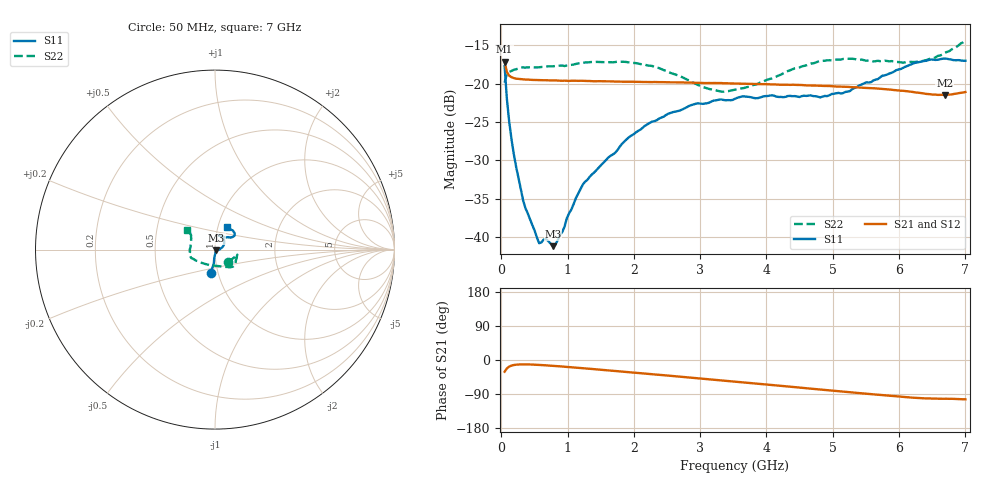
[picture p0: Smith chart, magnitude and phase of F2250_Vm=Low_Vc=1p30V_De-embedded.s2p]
! Integrated Device Technology
! Corporate Headquarters
! 6024 Silver Creek Valley Road
! San Jose, CA 95138  USA
! Phone:  1-408-284-8200
! Toll Free:  1-800-223-1366
! Webpage:  http://www.idt.com/
! Timing and RF Division
! 515 Groton Road, Suite 102
! Westford, MA 01886-6024
! Device:  F2250
! Description: Voltage Variable RF Attenuator
! Frequency:  50.0 -  6000.00 MHz
! Package:  3x3 mm Thin QFN Plastic Package: 16 pin
! Ports:  2 RF, 3 DC
!  Pin  1  = GND
!  Pin  2  = NC
!  Pin  3  = RF1  = Port 1
!  Pin  4  = NC
!  Pin  5  = GND
!  Pin  6  = GND
!  Pin  7  = GND
!  Pin  8  = GND
!  Pin  9  = NC
!  Pin 10  = RF2  = Port 2
!  Pin 11  = NC
!  Pin 12  = GND
!  Pin 13  = GND
!  Pin 14  = VCNTRL
!  Pin 15  = VDD
!  Pin 16  = VMODE
! Vcntrl:  1.300 Volts
! Vmode:  +0.000 Volts
! Vdd:  +3.30  Volts
! Current:  1.193 mA
! Data:  The device was measured on a the F2250 evaluation board which has
!  individual transmission lines to the RF pins.  Data was collected
!  using a calibrated network analyzer.  The evaluation board was
!  de-embedded using a TRL calibration technique.
!  The reference plane is the edge of the package pin.
! Misc:  SN 10
!  Action Tracker AT0258
! Date Measured:  2014-11-26
! Date:  2015-10-15  MJV
! Note:
!  Integrated Device Technology supplies this data as a sample of measured
!  data at the package pin for this product.  Your particular data for this
!  product may vary.
!  Data was taken at 25 degrees C.
!  Integrated Device Technology reserves the right to change this data at anytime.
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# GHz S dB R 50
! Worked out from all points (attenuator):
!   201 points, 50 MHz to 7 GHz, reference 50 ohm
!   highest |S21| = -17.15 dB at 50 MHz (marker M1); lowest = -21.5 dB at 6.687 GHz (marker M2)
!   lowest |S11| = -41.2 dB at 779.8 MHz (marker M3), VSWR 1.02, Z = 50.8 - j0.414 ohm
!   |S11| at or under -10 dB: start of sweep to end of sweep
!   |S22| runs from -21.1 to -14.4 dB; largest |S21 - S12| = 0.00035
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0.05  -17.72 -100.7  -17.15 -31.0  -17.15 -31.0  -19.87 -43.8
0.08475  -22.03 -95.0  -18.51 -22.0  -18.51 -22.0  -18.69 -21.6
0.15425  -27.25 -95.0  -19.17 -14.8  -19.18 -14.8  -18.36 -13.4
0.22375  -30.82 -90.0  -19.36 -12.4  -19.34 -12.4  -18.14 -12.7
0.328  -35.15 -81.7  -19.45 -11.5  -19.46 -11.5  -17.90 -12.9
0.57125  -40.77 -53.7  -19.54 -13.0  -19.56 -13.0  -17.88 -17.6
0.6755  -40.22 -44.6  -19.56 -14.1  -19.57 -14.1  -17.78 -20.0
0.77975  -41.15 -27.7  -19.58 -15.4  -19.58 -15.4  -17.75 -22.8
0.91875  -39.31 -15.1  -19.64 -17.2  -19.61 -17.2  -17.64 -26.7
0.98825  -37.53 -18.8  -19.64 -18.2  -19.64 -18.2  -17.64 -27.9
1.2315  -33.11 -2.2  -19.64 -21.6  -19.65 -21.6  -17.28 -32.9
1.9265  -26.96 19.8  -19.76 -32.1  -19.75 -32.1  -17.25 -43.6
2.37825  -24.56 30.8  -19.81 -39.0  -19.81 -39.0  -17.98 -51.5
2.86475  -22.80 45.4  -19.86 -46.7  -19.87 -46.7  -19.74 -67.0
3.14275  -22.45 53.2  -19.92 -51.1  -19.91 -51.1  -20.72 -82.3
3.525  -21.98 64.2  -19.99 -57.2  -19.99 -57.2  -20.78 -108.5
4.7065  -21.63 68.3  -20.26 -76.2  -20.26 -76.2  -17.36 -158.4
5.22775  -21.05 51.5  -20.43 -84.6  -20.44 -84.6  -16.78 -167.7
5.85325  -18.69 36.2  -20.78 -94.5  -20.78 -94.5  -17.10 179.2
6.33975  -17.13 38.1  -21.24 -100.8  -21.25 -100.8  -17.09 161.8
6.68725  -16.74 46.8  -21.49 -102.3  -21.49 -102.3  -16.01 148.3
7  -17.03 62.8  -21.09 -103.9  -21.09 -104.0  -14.39 145.0
